(* Logix 5000 Routine export Plant; software revision 20.01 *)

TYPE Key_Command :
STRUCT
   Command : SINT;
   Compliment : SINT;
   Arg_1 : SINT;
   Arg_2 : SINT;
END_STRUCT
END_TYPE

TYPE Freq_Output :
STRUCT
   Frequency : DINT;
   Status_Control : INT;
   Reserved : INT;
END_STRUCT
END_TYPE

TYPE MTB_Input :
STRUCT
   Digital_Out_Echo : INT;
   Analog_1_Echo : INT;
   Analog_2_Echo : INT;
   Status : INT;
   Channel : REAL[30];
   Speed : REAL;
   Ambient_Temperature : REAL;
   Digital_In : SINT;
END_STRUCT
END_TYPE

TYPE Plant :
STRUCT
   Slope_Load : REAL;
   Offset_Efficiency : REAL;
   Actuator_SteadyState : REAL;
   Actuator_Cur : REAL;
   TimeBase : TIMER;
   Actuator_Delta : REAL;
   Speed_Current : DINT;
   Accelleration : DINT;
   Speed_Output : DINT;
   Time_Multiplier : REAL;
   Direct_Frequency_Output : DINT;
   Manual_Actuator_Position : DINT;
   Freq_ComCode : INT;
   Freq_ComCount : INT;
   LoopCounter : COUNTER;
   Act_MTB_Voltage : REAL;
   Feedback_Pos : REAL;
   Update_Outputs : BOOL;
   Chan_Cfg : SINT;
   Speed_Status : SINT;
   Act_Status : SINT;
   Real1 : REAL;
   Real2 : REAL;
   DINT1 : DINT;
   DINT2 : DINT;
END_STRUCT
END_TYPE

TYPE Freq_Input :
STRUCT
   Comm_Status : INT;
   MODPlus_CPU_Usage : INT;
   Output_Frequency_Echo : DINT;
END_STRUCT
END_TYPE

TYPE GOVPlus_Input :
STRUCT
   Reserved1 : BOOL;
   Reserved2 : BOOL;
   V3_3Low : BOOL;
   V3_3High : BOOL;
   V5Low : BOOL;
   V5High : BOOL;
   V12_5Low : BOOL;
   V12_5High : BOOL;
   V24Low : BOOL;
   V24High : BOOL;
   AuxLoopLow : BOOL;
   AuxLoopHigh : BOOL;
   Reserved13 : BOOL;
   Reserved14 : BOOL;
   DemandLoopLow : BOOL;
   DemandLoopHigh : BOOL;
   CoolDownInputStatus : BOOL;
   StopInputStatus : BOOL;
   CurrentLoopOutputOpen : BOOL;
   SW1_Enabled_Echo : BOOL;
   SW1_Latching_Echo : BOOL;
   SW1_Failsafe_Echo : BOOL;
   Reserved23 : BOOL;
   Rotating : BOOL;
   AlarmOutActive : BOOL;
   StopOutClosed : BOOL;
   AuxOutputOutOfRange : BOOL;
   Target_Met : BOOL;
   Stop_Echo : BOOL;
   Reserved30 : BOOL;
   VoltOutActive : BOOL;
   V12_5SupplyFaulted : BOOL;
   Breaking : BOOL;
   WatchdogFailure : BOOL;
   FactoryCalEnabled : BOOL;
   WatchdogInhibited : BOOL;
   ActuatorEnabled : BOOL;
   Governing : BOOL;
   Timer1Active : BOOL;
   Timer2Active : BOOL;
   Timer3Active : BOOL;
   Purging : BOOL;
   Cooldown : BOOL;
   Max_Authority : BOOL;
   Demand_Active : BOOL;
   Target_Active : BOOL;
   Voltage_Driver_Output_On : BOOL;
   Reserved48 : BOOL;
   Aux_Output_Alarm : BOOL;
   Actuator_Output_Fault : BOOL;
   Overspeed : BOOL;
   Underspeed : BOOL;
   Stopped : BOOL;
   Reserved54 : BOOL;
   Reserved55 : BOOL;
   Reserved56 : BOOL;
   Reserved57 : BOOL;
   Reserved58 : BOOL;
   Reserved59 : BOOL;
   Reserved60 : BOOL;
   Reserved61 : BOOL;
   Reserved62 : BOOL;
   Reserved63 : BOOL;
   Reserved64 : BOOL;
   GovTime : REAL;
   Accelleration : REAL;
   RPM : DINT;
   RPMUnfiltered : REAL;
   DemandInput : REAL;
   AuxInput : REAL;
   CurrentOut : REAL;
   VoltageOut : REAL;
   Voltage_240 : REAL;
   Voltage_100 : REAL;
   Voltage_50 : REAL;
   Voltage_33 : REAL;
   Voltage_Output_Sense_Value : REAL;
   DemandTarget : DINT;
   ProcessorUsage : INT;
   GovState : INT;
   Speed_Target : REAL;
   Acceleration_Target : REAL;
   Acceleration_Error : REAL;
   RPM_Error : INT;
   Actuator_Position_Output : INT;
   ActuatorCounts : DINT;
   UpWindow : INT;
   DownWindow : INT;
   Float_Rsp : REAL;
   Comm_Status : INT;
   Spare_Echo : INT;
   Aux_Out_Echo : REAL;
END_STRUCT
END_TYPE

VAR_GLOBAL   (* controller tags *)
   GOV_Input : GOVPlus_Input := (SW1_Enabled_Echo := 1, SW1_Latching_Echo := 1, SW1_Failsafe_Echo := 1, Rotating := 1, StopOutClosed := 1, Target_Met := 1, Stop_Echo := 1, VoltOutActive := 1, WatchdogFailure := 1, ActuatorEnabled := 1, Governing := 1, Timer1Active := 1, Timer2Active := 1, Timer3Active := 1, Demand_Active := 1, Target_Active := 1, GovTime := 9.899902, Accelleration := -19.989746, RPM := 433, RPMUnfiltered := 413.57422, DemandInput := 18.0, AuxInput := 4.959961, CurrentOut := 5.329956, VoltageOut := 9.98999, Voltage_240 := 22.899902, Voltage_100 := 12.399902, Voltage_50 := 5.2999268, Voltage_33 := 3.1999512, Voltage_Output_Sense_Value := 9.899902, DemandTarget := 1800, ProcessorUsage := 37, GovState := 10, Speed_Target := 400.0, Acceleration_Target := -35.029297, Acceleration_Error := 15.039795, RPM_Error := 13, Actuator_Position_Output := 8, ActuatorCounts := 4276, UpWindow := 5, DownWindow := 5, Float_Rsp := 2.3999634, Comm_Status := 523, Aux_Out_Echo := 10.0);
   FreqGen_Input : Freq_Input := (MODPlus_CPU_Usage := 26, Output_Frequency_Echo := 467);
   MTB_Input : MTB_Input := (Digital_Out_Echo := 163, Analog_1_Echo := 256, Analog_2_Echo := 3604, Channel[0] := 302.0, Channel[1] := 299.0, Channel[4] := 6.34, Channel[5] := 1.0, Channel[7] := 3.95, Channel[10] := 1023.0, Channel[11] := 295.0, Channel[12] := 4.94, Channel[13] := 4002.0, Channel[14] := 1.27, Channel[15] := 1039.0, Channel[16] := 0.01, Channel[17] := 0.01, Channel[21] := 1.0, Channel[25] := -6.2, Channel[26] := -6.2, Channel[28] := 255.0, Channel[29] := 176.0, Speed := 386.0, Ambient_Temperature := 295.9);
   GOVPlus_Simulator : Plant := (Slope_Load := 15.0, Offset_Efficiency := 25.0, Actuator_SteadyState := 7380.0, Actuator_Cur := 6170.0, TimeBase.PRE := 100, Actuator_Delta := -1210.0, Speed_Current := 467, Accelleration := -81, Speed_Output := 459, Time_Multiplier := 0.1, Direct_Frequency_Output := 25, Manual_Actuator_Position := 4095, Act_MTB_Voltage := 9.88, Feedback_Pos := -24.9375, Update_Outputs := 1, Chan_Cfg := 2);
   GOV_KeyCommand : Key_Command := (Compliment := -7);
   GOV_KeyCommand_Msg : MESSAGE;
        MessageParameters(MessageType := CIP Generic, RequestedLength := 4, ConnectedFlag := 2, ConnectionPath := GOVPlus, ServiceCode := 16#004b, ObjectType := 16#006e, TargetObject := 1, LocalElement := GOV_KeyCommand)
   FreqGen_Output : Freq_Output := (Frequency := 467);
END_VAR

PROGRAM DET_COM

ROUTINE Plant   (* ladder *)
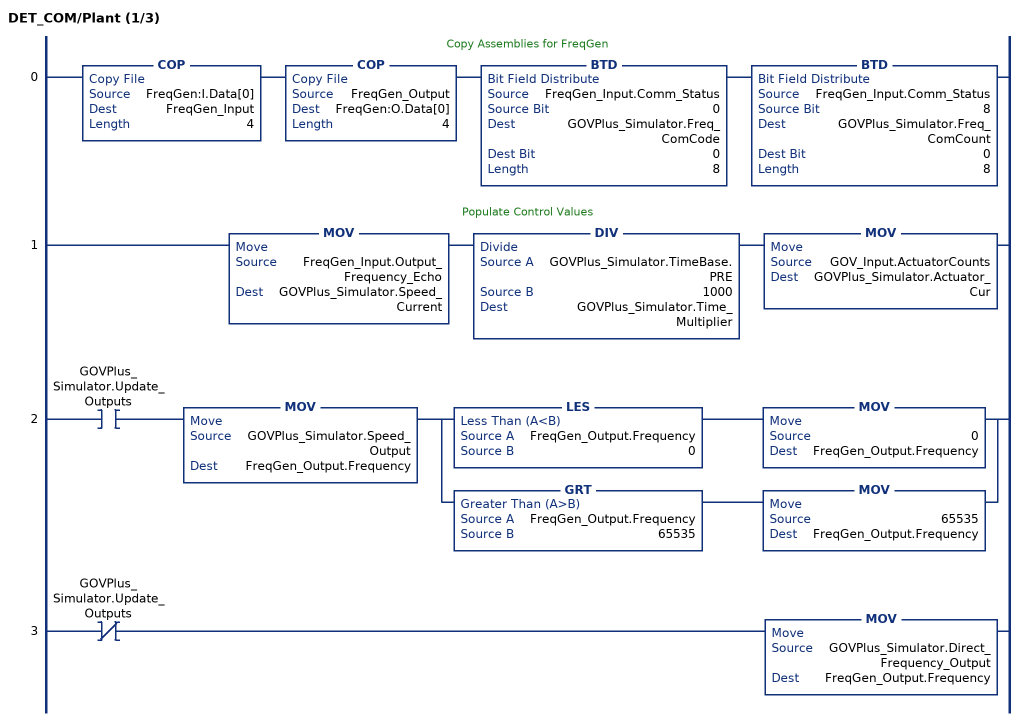
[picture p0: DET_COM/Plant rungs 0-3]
   // Copy Assemblies for FreqGen
   0: COP(FreqGen:I.Data[0],FreqGen_Input,4)COP(FreqGen_Output,FreqGen:O.Data[0],4)BTD(FreqGen_Input.Comm_Status,0,GOVPlus_Simulator.Freq_ComCode,0,8)BTD(FreqGen_Input.Comm_Status,8,GOVPlus_Simulator.Freq_ComCount,0,8);
   // Populate Control Values
   1: MOV(FreqGen_Input.Output_Frequency_Echo,GOVPlus_Simulator.Speed_Current)DIV(GOVPlus_Simulator.TimeBase.PRE,1000,GOVPlus_Simulator.Time_Multiplier)MOV(GOV_Input.ActuatorCounts,GOVPlus_Simulator.Actuator_Cur);
   2: XIC(GOVPlus_Simulator.Update_Outputs)MOV(GOVPlus_Simulator.Speed_Output,FreqGen_Output.Frequency)[LES(FreqGen_Output.Frequency,0) MOV(0,FreqGen_Output.Frequency) ,GRT(FreqGen_Output.Frequency,65535) MOV(65535,FreqGen_Output.Frequency) ];
   3: XIO(GOVPlus_Simulator.Update_Outputs)MOV(GOVPlus_Simulator.Direct_Frequency_Output,FreqGen_Output.Frequency);
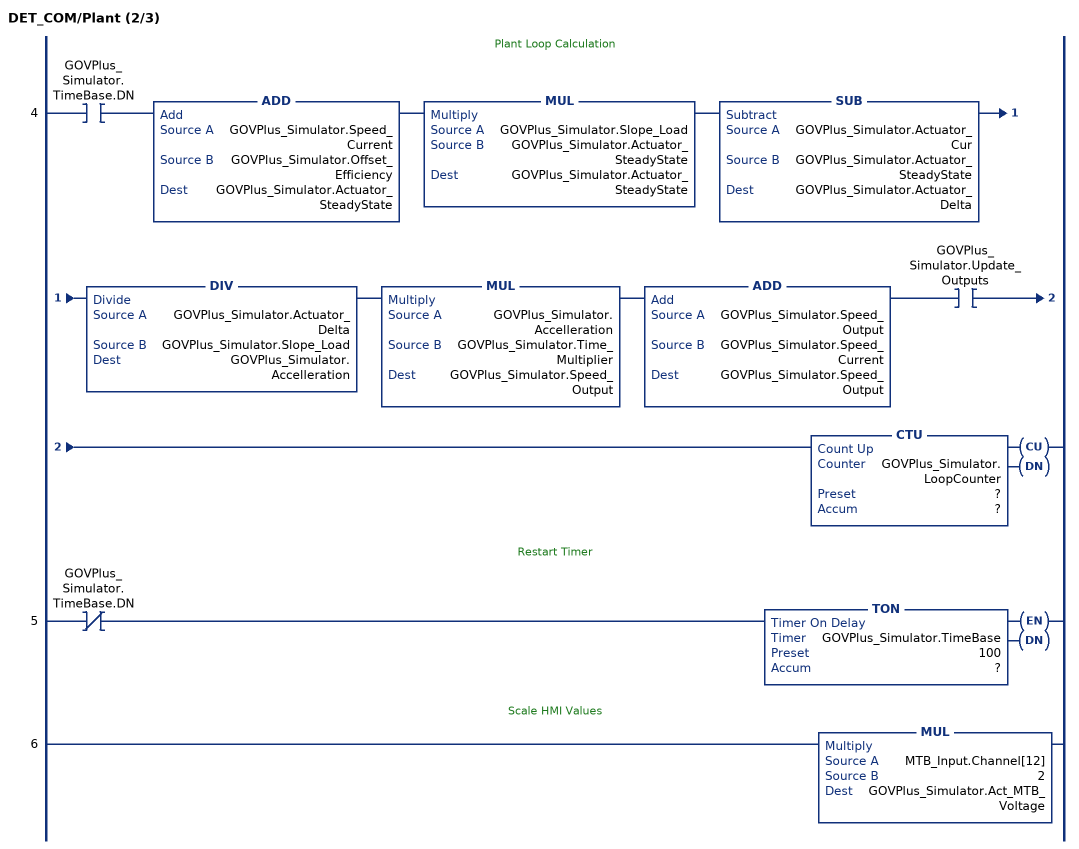
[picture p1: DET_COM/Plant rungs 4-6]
   // Plant Loop Calculation
   4: XIC(GOVPlus_Simulator.TimeBase.DN)ADD(GOVPlus_Simulator.Speed_Current,GOVPlus_Simulator.Offset_Efficiency,GOVPlus_Simulator.Actuator_SteadyState)MUL(GOVPlus_Simulator.Slope_Load,GOVPlus_Simulator.Actuator_SteadyState,GOVPlus_Simulator.Actuator_SteadyState)SUB(GOVPlus_Simulator.Actuator_Cur,GOVPlus_Simulator.Actuator_SteadyState,GOVPlus_Simulator.Actuator_Delta)DIV(GOVPlus_Simulator.Actuator_Delta,GOVPlus_Simulator.Slope_Load,GOVPlus_Simulator.Accelleration)MUL(GOVPlus_Simulator.Accelleration,GOVPlus_Simulator.Time_Multiplier,GOVPlus_Simulator.Speed_Output)ADD(GOVPlus_Simulator.Speed_Output,GOVPlus_Simulator.Speed_Current,GOVPlus_Simulator.Speed_Output)XIC(GOVPlus_Simulator.Update_Outputs)CTU(GOVPlus_Simulator.LoopCounter,?,?);
   // Restart Timer
   5: XIO(GOVPlus_Simulator.TimeBase.DN)TON(GOVPlus_Simulator.TimeBase,?,?);
   // Scale HMI Values
   6: MUL(MTB_Input.Channel[12],2,GOVPlus_Simulator.Act_MTB_Voltage);
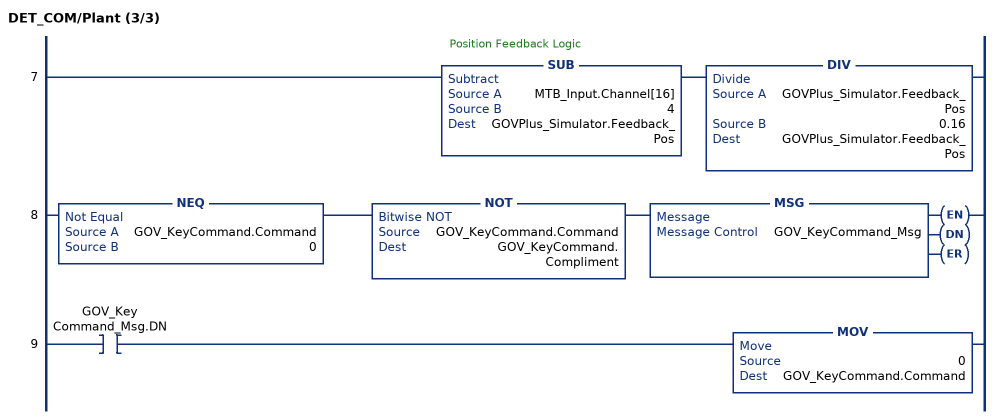
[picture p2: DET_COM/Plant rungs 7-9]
   // Position Feedback Logic
   7: SUB(MTB_Input.Channel[16],4,GOVPlus_Simulator.Feedback_Pos)DIV(GOVPlus_Simulator.Feedback_Pos,0.16,GOVPlus_Simulator.Feedback_Pos);
   8: NEQ(GOV_KeyCommand.Command,0)NOT(GOV_KeyCommand.Command,GOV_KeyCommand.Compliment)MSG(GOV_KeyCommand_Msg);
   9: XIC(GOV_KeyCommand_Msg.DN)MOV(0,GOV_KeyCommand.Command);
END_ROUTINE
END_PROGRAM
